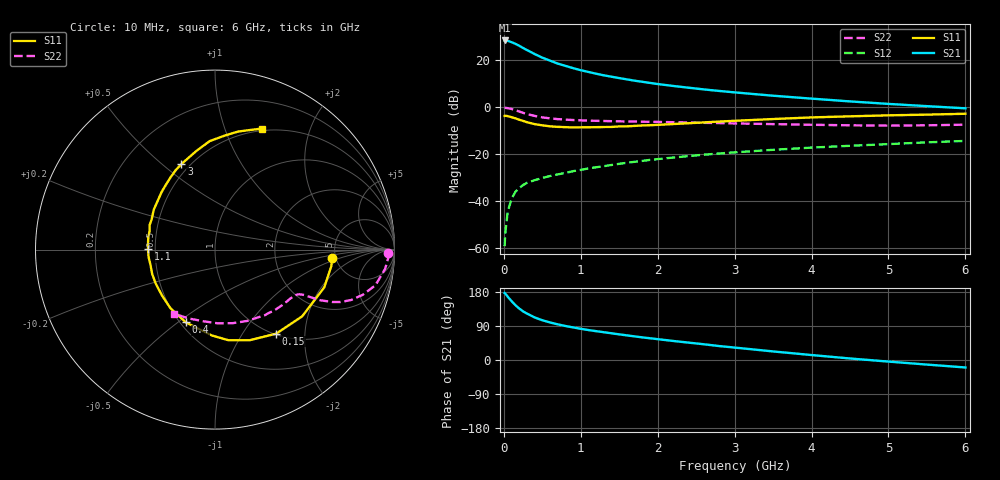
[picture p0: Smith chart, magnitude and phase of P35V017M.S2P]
! SIEMENS Small Signal Semiconductors
! BFP181
! Si NPN RF Bipolar Junction Transistor in SOT143
! VCE = 5 V  IC = 17 mA
! Common Emitter S-Parameters:  March  1996
# GHz  S  MA  R  50
!  f  S11  S21  S12  S22
! GHz  MAG  ANG  MAG  ANG  MAG  ANG  MAG  ANG
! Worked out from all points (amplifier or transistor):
!   36 points, 10 MHz to 6 GHz, reference 50 ohm
!   highest |S21| = 28.4 dB at 10 MHz (marker M1)
!   |S21| within 3 dB of that: start of sweep to 238.8 MHz
!   unconditionally stable (mu >= 1): 847.2 MHz to 5.997 GHz
!   at 250 MHz: K = 0.45, MSG = 29.2 dB, |S12| = -33.2 dB
!   at 1.4 GHz: K = 1.16, MAG = 16.3 dB, |S12| = -24.6 dB
!   at 6 GHz: K = 1.00, MSG = 6.9 dB, |S12| = -14.4 dB
!   S11 on the Smith chart (normalised r, x): 10 MHz: 4.63, -0.71; 150 MHz: 1.02, -1.43; 400 MHz: 0.53, -0.53; 1.1 GHz: 0.46, +0.00; 3 GHz: 0.45, +0.58; 6 GHz: 0.48, +1.35
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0.01  0.652 -3.9  26.29 176.8  0.0011 80.6  0.9656 -1.0
0.02  0.6551 -7.9  26.24 174.9  0.0022 83.1  0.9677 -2.4
0.05  0.6442 -19.1  25.84 167.1  0.0059 80.8  0.9537 -6.5
0.1  0.6115 -37.5  24.16 155.4  0.0112 71.8  0.9159 -12.5
0.15  0.5794 -53.9  22.29 144.7  0.0158 66.1  0.8613 -17.0
0.2  0.5405 -69.1  20.26 135.8  0.019 63.6  0.8072 -20.4
0.25  0.5104 -81.6  18.16 128.3  0.022 59.3  0.7568 -22.7
0.3  0.4785 -92.2  16.45 122.6  0.0245 57.2  0.7148 -24.1
0.4  0.4366 -111.9  13.53 112.3  0.0279 54.2  0.6511 -25.7
0.5  0.4104 -127.2  11.31 104.9  0.0311 52.8  0.6067 -26.3
0.6  0.3912 -138.7  9.78 99.1  0.0342 53.3  0.5779 -26.7
0.7  0.381 -149.7  8.468 94.1  0.0371 53.5  0.5572 -27.0
0.9  0.3695 -166.2  6.775 86.0  0.0434 53.6  0.532 -27.9
1.1  0.3733 179.7  5.611 79.0  0.0497 54.1  0.5168 -29.3
1.3  0.3781 169.1  4.757 73.3  0.0556 54.3  0.5076 -31.2
1.6  0.3908 154.8  3.899 65.0  0.0657 53.6  0.4965 -34.6
2.2  0.4371 133.0  2.83 50.3  0.0846 50.9  0.4781 -42.9
3  0.5122 111.4  2.064 32.8  0.1093 45.4  0.4503 -56.2
3.5  0.5588 100.8  1.752 22.6  0.1237 41.7  0.4359 -65.8
4.5  0.6382 85.0  1.326 4.0  0.1507 33.4  0.4109 -87.9
5.5  0.6936 73.8  1.051 -12.1  0.1782 26.1  0.411 -111.1
6  0.724 68.7  0.945 -19.7  0.1913 21.9  0.4242 -122.9
